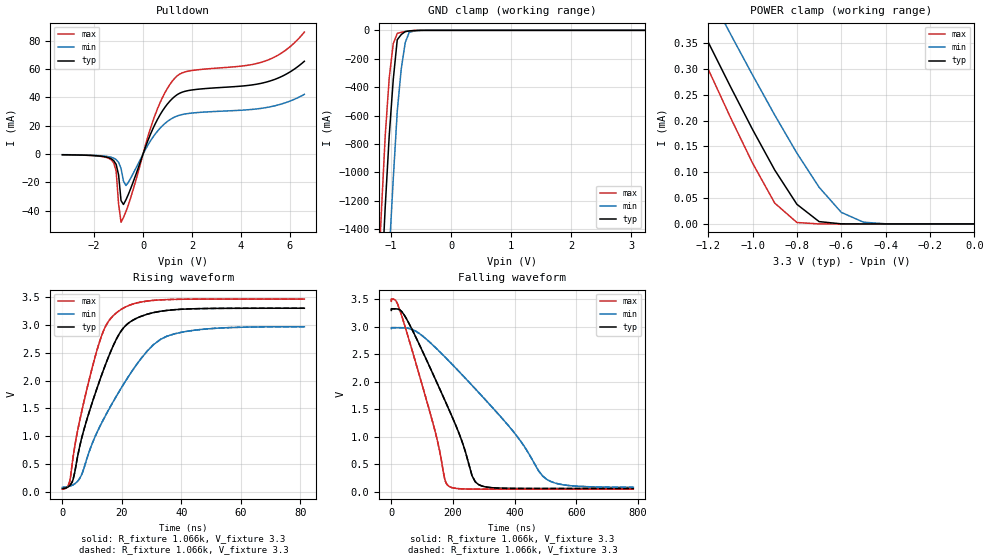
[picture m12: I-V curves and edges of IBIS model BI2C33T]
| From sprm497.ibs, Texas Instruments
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|   Model Cell BI2C33T
|BI2C33T
[Model]   BI2C33T
Model_type   I/O_open_drain
Polarity   Non-Inverting
Enable   Active-Low
Vinl =  0.99
Vinh =  2.31
Cref =  400pF
Rref =  528
Vref =  1.8V
Vmeas =  1.65
C_comp   5.331859p   4.20754p   6.280885p
[Model Spec]
Vinl   0.99   0.891   1.0395
Vinh   2.31   2.079   2.4255
[Temperature Range]   25   125   -40
[Voltage Range]   3.3   2.97   3.465
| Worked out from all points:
|   slope of the pulldown table from 0 to 0.495 V, typ, clamps not added: 23.3 ohm
|   GND clamp passes 1 mA (typ) near -0.58 V on its own axis
|   POWER clamp passes 1 mA (typ) near -1.93 V on its own axis
|   rising waveform, R_fixture 1.066k, V_fixture 3.3: 20-80 % time 11.9ns typ, 17.8ns min, 9.11ns max; typ from 0.06 V to 3.3 V
|   rising waveform, R_fixture 1.066k, V_fixture 3.3: 20-80 % time 11.9ns typ, 17.8ns min, 9.11ns max; typ from 0.06 V to 3.3 V
|   falling waveform, R_fixture 1.066k, V_fixture 3.3: 20-80 % time 148ns typ, 265ns min, 101ns max; typ from 3.3 V to 0.06 V
|   falling waveform, R_fixture 1.066k, V_fixture 3.3: 20-80 % time 148ns typ, 265ns min, 101ns max; typ from 3.3 V to 0.06 V
[POWER_clamp]
|   voltage   I(typ)   I(min)   I(max)
-3.3V     2.258mA    2.24mA     2.38mA
-1.3V     439.3uA    531.8uA    394.9uA
-1.267V   410.2uA    504.3uA    363.1uA
-1.233V   381.1uA    476.9uA    331.4uA
-1.133V   294.8uA    395.3uA    237.6uA
-1.1V     266.2uA    368.2uA    206.6uA
-900mV    104.4uA    210.8uA    40.39uA
-800mV    37.97uA    137.1uA    2.806uA
-700mV    4.533uA    71.05uA    36.21nA
-600mV    182.6nA    22.43uA    335.5pA
-500mV    4.782nA    3.391uA    31.36pA
-11.55fV  253pA      12.31nA    13.46pA
[Pulldown]
|   voltage   I(typ)   I(min)   I(max)
-3.3V     -494.3uA   -432.4uA   -501.7uA
-1.3V     -3.369mA   -2.303mA   -4.135mA
-1.1V     -7.33mA    -3.923mA   -12.08mA
-1V       -14.76mA   -5.85mA    -35.39mA
-900mV    -32.93mA   -10.24mA   -48.19mA
-800mV    -35.66mA   -19.12mA   -44.87mA
-700mV    -32.38mA   -22.28mA   -40.77mA
500mV     21.44mA    14.19mA    28mA
1.3V      40.76mA    26.23mA    53.69mA
1.9V      45.03mA    28.79mA    58.77mA
5V        50.69mA    32.76mA    65.78mA
6.6V      65.62mA    42.22mA    86.24mA
[GND_clamp]
|   voltage   I(typ)   I(min)   I(max)
-3.3V     -22.49A    -23.29A    -22.05A
-1.233V   -2.406A    -3.298A    -1.884A
-1.167V   -1.816A    -2.702A    -1.3A
-1.1V     -1.241A    -2.115A    -739mA
-1.033V   -739mA     -1.563A    -333.4mA
-966.7mV  -347.4mA   -1.048A    -94.19mA
-900mV    -66.29mA   -570.3mA   -21.26mA
-833.3mV  -29.57mA   -271.1mA   -14.09mA
-766.7mV  -8.918mA   -85.58mA   -8.243mA
-700mV    -4.339mA   -13.71mA   -3.72mA
-433.3mV  -62.98uA   -247.3uA   -19.28uA
3.233V    237.5pA    29.91nA    9.237pA
[Ramp]
| variable   typ   min   max
dV/dt_f   1.961066/0.149772u   1.74288/0.2669127u   2.074494/0.1019836u
dV/dt_r  82.35656m/1.72526n   57.20466m/4.0595n   98.88726m/1.019786n
R_load = 1.066k
[Rising Waveform]
R_fixture = 1.066k
V_fixture = 3.3
V_fixture_min = 2.97
V_fixture_max = 3.465
|   time   V(typ)   V(min)   V(max)
0s        60.23mV    81mV       48.5mV
2.4ns     108.1mV    101.2mV    172.6mV
3.6ns     221.7mV    127.6mV    623.8mV
6.6ns     991mV      325.3mV    1.47V
12ns      1.917V     1.11V      2.613V
14.7ns    2.317V     1.392V     2.994V
18.3ns    2.761V     1.734V     3.224V
23.7ns    3.086V     2.194V     3.376V
35.1ns    3.261V     2.797V     3.455V
81.3ns    3.3V       2.967V     3.465V
[Rising Waveform]
R_fixture = 1.066k
V_fixture = 3.3
V_fixture_min = 2.97
V_fixture_max = 3.465
|   time   V(typ)   V(min)   V(max)
0s        60.23mV    81mV       48.5mV
2.4ns     108.1mV    101.2mV    172.6mV
3.6ns     221.7mV    127.6mV    623.8mV
6.6ns     991mV      325.3mV    1.47V
12ns      1.917V     1.11V      2.613V
14.7ns    2.317V     1.392V     2.994V
18.3ns    2.761V     1.734V     3.224V
23.7ns    3.086V     2.194V     3.376V
35.1ns    3.261V     2.797V     3.455V
81.3ns    3.3V       2.967V     3.465V
[Falling Waveform]
R_fixture = 1.066k
V_fixture = 3.3
V_fixture_min = 2.97
V_fixture_max = 3.465
|   time   V(typ)   V(min)   V(max)
0s        3.3V       2.97V      3.465V
14.1ns    3.328V     2.986V     3.483V
41.1ns    3.222V     2.983V     3.068V
143.1ns   2.043V     2.623V     1.074V
173.4ns   1.666V     2.455V     224.5mV
186ns     1.507V     2.383V     103.9mV
261.6ns   293.8mV    1.937V     49.88mV
292.8ns   107.6mV    1.748V     48.87mV
504.9ns   60.33mV    222.6mV    48.5mV
784.5ns   60.23mV    83.97mV    48.5mV
[Falling Waveform]
R_fixture = 1.066k
V_fixture = 3.3
V_fixture_min = 2.97
V_fixture_max = 3.465
|   time   V(typ)   V(min)   V(max)
0s        3.3V       2.97V      3.465V
14.1ns    3.328V     2.986V     3.483V
41.1ns    3.222V     2.983V     3.068V
143.1ns   2.043V     2.623V     1.074V
173.4ns   1.666V     2.455V     224.5mV
186ns     1.507V     2.383V     103.9mV
261.6ns   293.8mV    1.937V     49.88mV
292.8ns   107.6mV    1.748V     48.87mV
504.9ns   60.33mV    222.6mV    48.5mV
784.5ns   60.23mV    83.97mV    48.5mV
